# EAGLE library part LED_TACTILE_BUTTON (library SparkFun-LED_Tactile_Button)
LED Tactile Button Device for SparkFun Electronics' LED Tactile Button. In part derived from BOB-10467 - LED Tactile Button Breakout. Released under the Creative Commons Attribution Share-Alike 3.0 License http://creativecommons.org/licenses/by-sa/3.0 COM-10439 - White COM-10440 - Green COM-10441 - Orange COM-10442 - Red COM-10443 - Blue
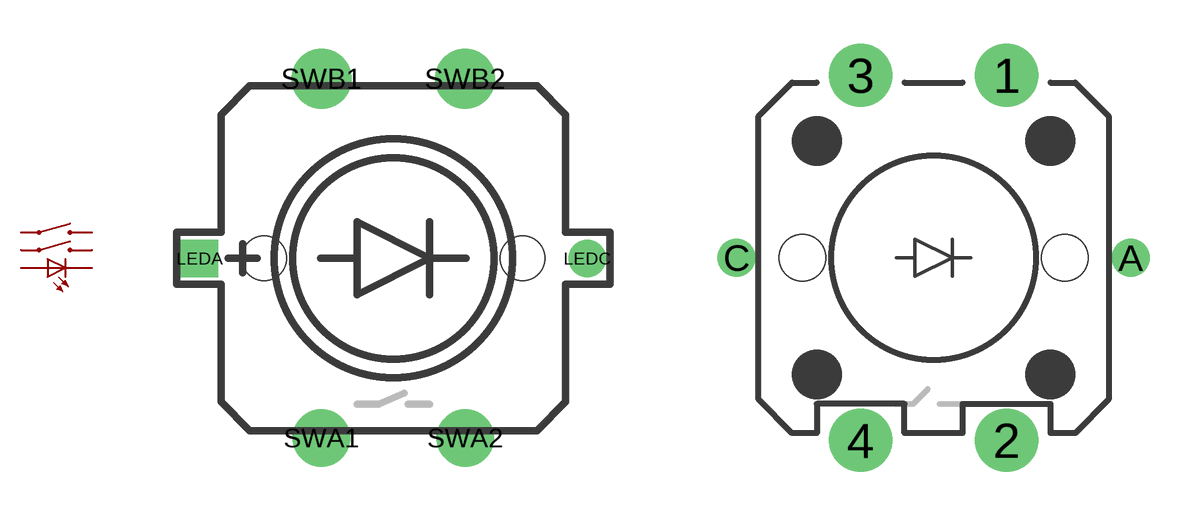
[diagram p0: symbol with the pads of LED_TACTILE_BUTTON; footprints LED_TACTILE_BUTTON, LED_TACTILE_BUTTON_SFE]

Designator prefix LSW

## LED_TACTILE_BUTTON  [LED_TACTILE_BUTTON]
LEDA  LEDA  pas
LEDC  LEDC  pas
SWA1  SWA1  pas
SWA2  SWA2  pas
SWB1  SWB1  pas
SWB2  SWB2  pas

## LED_TACTILE_BUTTONSFE  [LED_TACTILE_BUTTON_SFE]
1  SWB2  pas
2  SWA2  pas
3  SWB1  pas
4  SWA1  pas
A  LEDA  pas
C  LEDC  pas

## Footprint LED_TACTILE_BUTTON (pad centres in mm)
LED Tactile Button Package for SparkFun Electronics' LED Tactile Button.
drill 0.8 square: LEDA -6.75,0
drill 0.8: LEDC 6.75,0
drill 1.2 pad 2: SWA1 -2.5,-6.25; SWA2 2.5,-6.25
drill 1.2 pad 2.1: SWB1 -2.5,6.25; SWB2 2.5,6.25
hole 1.55 at -4.5,0
hole 1.55 at 4.5,0

## Footprint LED_TACTILE_BUTTON_SFE (pad centres in mm)
LED Tactile Button Package for SparkFun Electronics' LED Tactile Button. Derived from BOB-10467 - LED Tactile Button Breakout. Released under the Creative Commons Attribution Share-Alike 3.0 License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
drill 1.2 pad 2.159: 1 2.5,6.25; 2 2.5,-6.25; 3 -2.5,6.25; 4 -2.5,-6.25
drill 0.8: A 6.75,0; C -6.75,0
hole 1.6 at 4.5,0
hole 1.6 at -4.5,0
